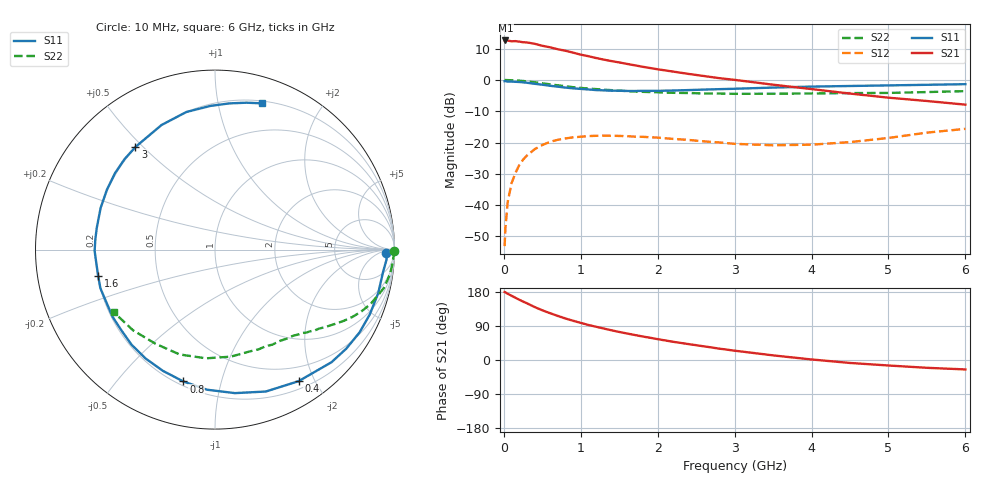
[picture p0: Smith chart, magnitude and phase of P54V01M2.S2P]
! SIEMENS Small Signal Semiconductors
! BFP183
! Si NPN RF Bipolar Junction Transistor in SOT143
! VCE = 4 V  IC = 1.2 mA
! Common Emitter S-Parameters:  March  1996
# GHz  S  MA  R  50
!  f  S11  S21  S12  S22
! GHz  MAG  ANG  MAG  ANG  MAG  ANG  MAG  ANG
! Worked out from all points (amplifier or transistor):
!   36 points, 10 MHz to 6 GHz, reference 50 ohm
!   highest |S21| = 12.6 dB at 20 MHz (marker M1)
!   |S21| within 3 dB of that: start of sweep to 741.1 MHz
!   unconditionally stable (mu >= 1): 2.43 GHz to end of sweep
!   at 250 MHz: K = 0.10, MSG = 18.8 dB, |S12| = -25.5 dB
!   at 1.4 GHz: K = 0.56, MSG = 11.9 dB, |S12| = -17.8 dB
!   at 6 GHz: K = 1.00, MAG = 3.5 dB, |S12| = -15.6 dB
!   S11 on the Smith chart (normalised r, x): 10 MHz: 35, -17; 400 MHz: 0.30, -1.78; 800 MHz: 0.22, -0.76; 1.6 GHz: 0.20, -0.11; 3 GHz: 0.20, +0.47; 6 GHz: 0.22, +1.35
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0.01  0.9553 -1.3  4.203 179.3  0.0022 87.6  0.9999 -0.5
0.02  0.9578 -3.2  4.283 178.5  0.0042 81.3  0.9973 -1.0
0.05  0.9446 -7.6  4.269 174.8  0.0112 85.6  0.9945 -2.6
0.1  0.9412 -14.9  4.151 169.6  0.0223 80.4  0.9901 -5.2
0.15  0.9351 -22.7  4.179 164.3  0.0325 76.3  0.9844 -7.9
0.2  0.9282 -29.8  4.106 159.2  0.0433 72.6  0.9738 -10.4
0.3  0.9029 -44.0  3.984 149.7  0.0619 64.2  0.9478 -15.0
0.4  0.8685 -57.6  3.79 139.8  0.0781 56.4  0.9181 -19.3
0.5  0.8399 -70.3  3.519 131.2  0.0912 49.5  0.8846 -23.0
0.6  0.8073 -82.1  3.33 123.6  0.1024 43.4  0.8526 -26.1
0.8  0.7555 -103.5  2.932 109.6  0.1161 32.9  0.7933 -31.2
0.9  0.7353 -113.2  2.734 103.6  0.1209 28.4  0.767 -33.5
1.1  0.705 -131.2  2.397 92.4  0.1267 20.8  0.728 -37.2
1.4  0.6728 -154.0  2.003 78.4  0.1283 11.7  0.6872 -42.3
1.6  0.6673 -167.3  1.809 70.0  0.1265 7.5  0.6649 -45.2
1.8  0.6707 -179.4  1.63 62.2  0.1233 4.3  0.646 -48.3
2.2  0.6783 159.9  1.362 48.1  0.1142 -0.5  0.623 -55.0
3  0.7234 127.8  1.004 24.6  0.0952 -0.2  0.5999 -70.6
3.5  0.7555 113.2  0.84 12.2  0.0903 6.5  0.6029 -81.6
4.5  0.801 91.8  0.606 -7.8  0.1015 21.6  0.6165 -108.7
5.5  0.837 77.9  0.461 -20.6  0.1438 26.4  0.6407 -135.4
6  0.8563 72.1  0.403 -24.9  0.1654 23.4  0.6627 -148.1
